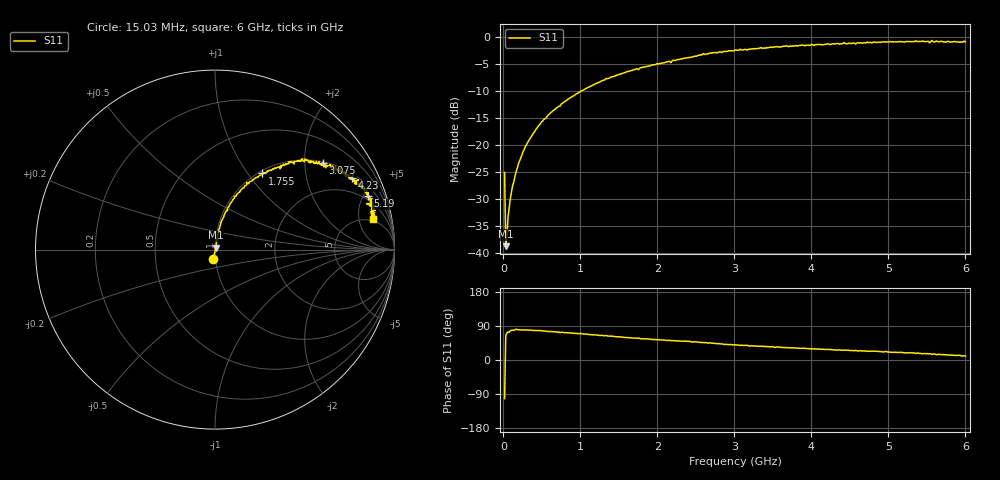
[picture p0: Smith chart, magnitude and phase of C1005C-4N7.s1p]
!	Network	Analyzer	HP8753E.07.74:	Oct	30	2002	Serial	No.	JP38451487
!	Hewlett-Packard
!	7	Sep	2009	8:26:39
!	Frequency	S11
#	HZ	S	RI	R	50
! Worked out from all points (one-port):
!   400 points, 15.03 MHz to 6 GHz, reference 50 ohm
!   lowest |S11| = -38.7 dB at 30.03 MHz (marker M1), VSWR 1.02, Z = 50.5 + j1.05 ohm
!   |S11| at or under -10 dB: start of sweep to 1.008 GHz
!   S11 on the Smith chart (normalised r, x): 15.03 MHz: 0.97, -0.11; 1.755 GHz: 1.04, +1.17; 3.075 GHz: 1.04, +2.47; 4.23 GHz: 1.22, +3.71; 5.19 GHz: 1.70, +5.35; 6 GHz: 4.49, +7.98
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1.502992e7  -0.0116 -0.0544
3.002985e7  0.00506 0.0104
4.502978e7  0.00471 0.014
6.00297e7  0.00595 0.0209
1.050295e8  0.00755 0.0364
1.95029e8  0.0117 0.0664
2.550287e8  0.0161 0.0852
4.950275e8  0.0354 0.16
7.650262e8  0.0702 0.233
1.095025e9  0.129 0.315
1.515022e9  0.22 0.394
1.755021e9  0.262 0.424
2.265019e9  0.393 0.478
3.015015e9  0.581 0.49
3.075015e9  0.603 0.481
3.165014e9  0.588 0.474
3.765011e9  0.696 0.438
4.230009e9  0.763 0.397
4.515007e9  0.788 0.369
4.965005e9  0.827 0.346
5.190004e9  0.85 0.298
5.265004e9  0.859 0.292
5.445003e9  0.882 0.258
5.535002e9  0.845 0.255
5.565002e9  0.897 0.241
5.595002e9  0.862 0.245
5.625002e9  0.893 0.217
6e9  0.883 0.17
